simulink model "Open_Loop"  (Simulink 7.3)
settings: Solver=ode45  StartTime=0.0  StopTime=30  RelTol=1e-3
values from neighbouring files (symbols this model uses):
  d2r = pi/180    (= 0.0174532925199)    [start.m]    (also in Pl.m; run.m; pl.m)
  Ka = (1+2*zeta*lamb)*Jgi*wcmg^2    (= 292500)    [start.m]
  Kb = (2*zeta+lamb)*wcmg/Ka    (= 0.00410256410256)    [start.m]
  ki = 0.07    [start.m]
  Kii = lamb*Jgi*wcmg^3    (= 37500000)    [start.m]
  kp = 7.3    [start.m]
  r2d = 180/pi    (= 57.2957795131)    [start.m]    (also in Pl.m; run.m; pl.m)
undefined symbols (not defined in the file or in its folder): Af, Bf, Cf, Df, Lin_Steering, Tglim

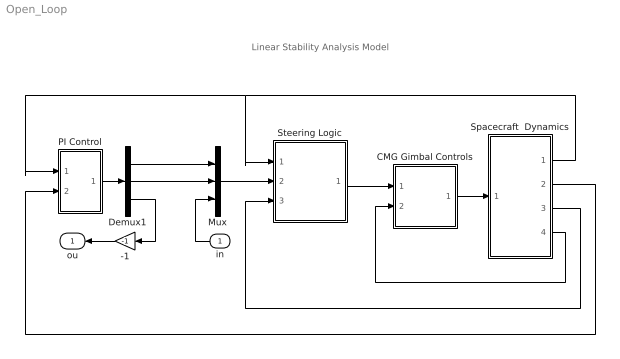
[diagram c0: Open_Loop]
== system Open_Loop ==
  note: Linear Stability Analysis Model
  in : Inport
  -1 : Gain  Gain=-1  ParameterDataType=sfix(16)  ParameterScaling=2^0  OutDataType=sfix(16)  OutScaling=2^0
  CMG Gimbal Controls : Subsystem
  Demux1 : Demux  Outputs=3
  Mux : Mux  Inputs=3
  PI Control : Subsystem
  Spacecraft  Dynamics : Subsystem
  Steering Logic : Subsystem
  ou : Outport
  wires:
  CMG Gimbal Controls/1(Tc) -> Spacecraft  Dynamics/1(Tc)
  Spacecraft  Dynamics/4(deldot) -> CMG Gimbal Controls/2(deldot)
  Steering Logic/1(deldot) -> CMG Gimbal Controls/1(deldc)
  Spacecraft  Dynamics/1(rate) -> Steering Logic/1(wb), PI Control/1(wb)
  Spacecraft  Dynamics/3(delta) -> Steering Logic/3(delta)
  Spacecraft  Dynamics/2(atti) -> PI Control/2(ater)
  Mux/1 -> Steering Logic/2(we)
  PI Control/1(wer) -> Demux1/1
  -1/1 -> ou/1
  Demux1/1 -> Mux/1
  Demux1/2 -> Mux/2
  Demux1/3 -> -1/1
  in/1 -> Mux/3

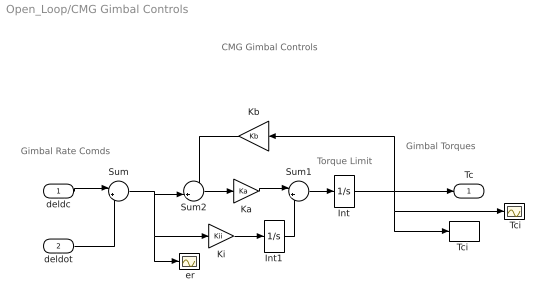
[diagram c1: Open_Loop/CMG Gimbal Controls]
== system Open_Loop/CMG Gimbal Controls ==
  note: Gimbal Rate Comds
  note: CMG Gimbal Controls
  note: Torque Limit
  note: Gimbal Torques
  deldc : Inport  PortDimensions=4  OutDataType=sfix(16)  OutScaling=2^0
  deldot : Inport  Port=2  PortDimensions=4  OutDataType=sfix(16)  OutScaling=2^0
  " Tci" : Scope
  " er" : Scope
  Int : Integrator  UpperSaturationLimit=[1 1 1 1]*Tglim  LowerSaturationLimit=-[1 1 1 1]*Tglim
  Int1 : Integrator  UpperSaturationLimit=0  LowerSaturationLimit=0
  Ka : Gain  Gain=Ka  ParameterDataType=sfix(16)  ParameterScaling=2^0  OutDataType=sfix(16)  OutScaling=2^0
  Kb : Gain  Gain=Kb  ParameterDataType=sfix(16)  ParameterScaling=2^0  OutDataType=sfix(16)  OutScaling=2^0
  Ki : Gain  Gain=Kii  ParameterDataType=sfix(16)  ParameterScaling=2^0  OutDataType=sfix(16)  OutScaling=2^0
  Sum : Sum  Inputs=|+-  OutDataType=sfix(16)  OutScaling=2^0
  Sum1 : Sum  Inputs=|++  OutDataType=sfix(16)  OutScaling=2^0
  Sum2 : Sum  Inputs=-+|  OutDataType=sfix(16)  OutScaling=2^0
  "Tci " : ToWorkspace  VariableName=Tci  SampleTime=-1  SaveFormat=Array
  Tc : Outport  OutDataType=sfix(16)  OutScaling=2^0
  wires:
  deldot/1 -> Sum/2
  deldc/1 -> Sum/1
  Sum/1 -> " er"/1, Ki/1, Sum2/2
  Kb/1 -> Sum2/1
  Int1/1 -> Sum1/2
  Ki/1 -> Int1/1
  Sum1/1 -> Int/1
  Ka/1 -> Sum1/1
  Sum2/1 -> Ka/1
  Int/1 -> Tc/1, " Tci"/1, "Tci "/1, Kb/1

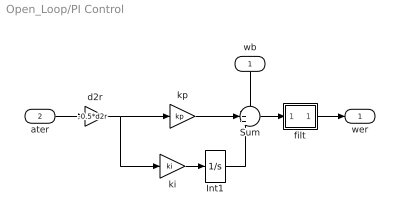
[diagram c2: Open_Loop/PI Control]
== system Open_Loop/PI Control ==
  wb : Inport
  ater : Inport  Port=2
  Int1 : Integrator  UpperSaturationLimit=0  LowerSaturationLimit=0
  Sum : Sum  Inputs=-++  OutDataType=sfix(16)  OutScaling=2^0
  d2r : Gain  Gain=-0.5*d2r  ParameterDataType=sfix(16)  ParameterScaling=2^0  OutDataType=sfix(16)  OutScaling=2^0
  filt : Subsystem
  ki : Gain  Gain=ki  ParameterDataType=sfix(16)  ParameterScaling=2^0  OutDataType=sfix(16)  OutScaling=2^0
  kp : Gain  Gain=kp  ParameterDataType=sfix(16)  ParameterScaling=2^0  OutDataType=sfix(16)  OutScaling=2^0
  wer : Outport
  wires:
  ater/1 -> d2r/1
  kp/1 -> Sum/2
  ki/1 -> Int1/1
  Int1/1 -> Sum/3
  wb/1 -> Sum/1
  Sum/1 -> filt/1(in)
  d2r/1 -> ki/1, kp/1
  filt/1(ou) -> wer/1

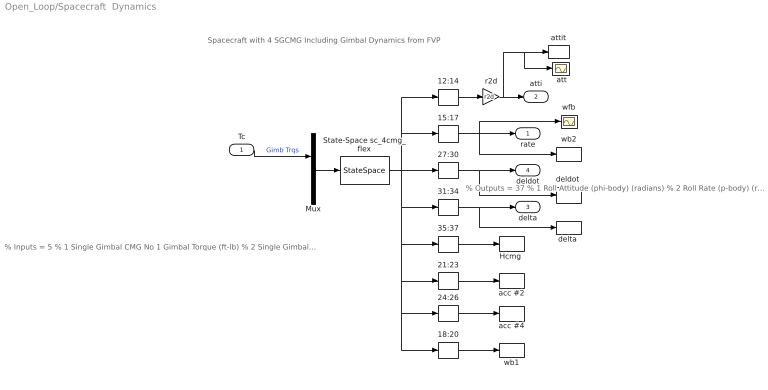
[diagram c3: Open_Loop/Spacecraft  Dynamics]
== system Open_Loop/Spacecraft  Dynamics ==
  note: % Outputs = 37 % 1 Roll Attitude (phi-body) (radians) % 2 Roll Rate (p-body) (rad/sec) % 3 Pitch Attitude (thet-bdy) (radians) % 4 Pitch Rate (q-body) (rad/sec) % 5 Yaw Attitude (psi-body) (radians) % 6 Yaw Rate (r-body) (rad/sec) % 7 Angle of attack, alfa, (radians) % 8 Angle of sideslip, beta, (radian) % 9 Change in Altitude, delta-h, (feet) % 10 Forward Acceleration (V-dot) (ft/sec) % 11 Cross Range Velocity (Vcr) (ft/sec) % 12 Gyro # 1, Roll Attitude (Body) (radians) % 13 Gyro # 2, Pitch Attitude (Body) (radians) % 14 Gyro # 3, Yaw Attitude (Body) (radians) % 15 Rate-Gyro # 4, Roll Rate (Body) (rad/sec) % 16 Rate-Gyro # 5, Pitch Rate (Body) (rad/sec) % 17 Rate-Gyro # 6, Yaw Rate (Body) (rad/sec) % 18 Rate-Gyro # 7, Roll Rate (Body) (rad/sec) % 19 Rate-Gyro # 8, Pitch Rate (Body) (rad/sec) % 20 Rate-Gyro # 9, Yaw Rate (Body) (rad/sec) % 21 Accelerom # 1, (along X), (ft/sec^2) Translat. Acceler % 22 Accelerom # 2, (along Y), (ft/sec^2) Translat. Acceler % 23 Accelerom # 3, (along Z), (ft/sec^2) Translat. Acceler % 24 Accelerom # 4, (along X), (ft/sec^2) Translat. Acceler % 25 Accelerom # 5, (along Y), (ft/sec^2) Translat. Acceler % 26 Accelerom # 6, (along Z), (ft/sec^2) Translat. Acceler % 27 SGCMG # 1 Gimbal Rate (rad/sec) % 28 SGCMG # 2 Gimbal Rate (rad/sec) % 29 SGCMG # 3 Gimbal Rate (rad/sec) % 30 SGCMG # 4 Gimbal Rate (rad/sec) % 31 SGCMG # 1 Gimbal Angle (radian) % 32 SGCMG # 2 Gimbal Angle (radian) % 33 SGCMG # 3 Gimbal Angle (radian) % 34 SGCMG # 4 Gimbal Angle (radian) % 35 SGCMG Array Momentum in X-axis (ft-lb-sec) % 36 SGCMG Array Momentum in Y-axis (ft-lb-sec) % 37 SGCMG Array Momentum in Z-axis (ft-lb-sec)
  note: % Inputs = 5 % 1 Single Gimbal CMG No 1 Gimbal Torque (ft-lb) % 2 Single Gimbal CMG No 2 Gimbal Torque (ft-lb) % 3 Single Gimbal CMG No 3 Gimbal Torque (ft-lb) % 4 Single Gimbal CMG No 4 Gimbal Torque (ft-lb) % 5 Ext Force Direct. = (1.0000 0.0000 0.0000)
  note: Spacecraft with 4 SGCMG Including Gimbal Dynamics from FVP
  Tc : Inport  PortDimensions=4  OutDataType=sfix(16)  OutScaling=2^0
  " att" : Scope
  " wfb " : Scope
  12:14 : Selector  InputPortWidth=37  IndexOptions=Index vector (dialog)  Indices=[12:14]  OutputSizes=1
  15:17 : Selector  InputPortWidth=37  IndexOptions=Index vector (dialog)  Indices=[15:17]  OutputSizes=1
  18:20 : Selector  InputPortWidth=37  IndexOptions=Index vector (dialog)  Indices=[18:20]  OutputSizes=1
  21:23 : Selector  InputPortWidth=37  IndexOptions=Index vector (dialog)  Indices=[21:23]  OutputSizes=1
  24:26 : Selector  InputPortWidth=37  IndexOptions=Index vector (dialog)  Indices=[24:26]  OutputSizes=1
  27:30 : Selector  InputPortWidth=37  IndexOptions=Index vector (dialog)  Indices=[27:30]  OutputSizes=1
  31:34 : Selector  InputPortWidth=37  IndexOptions=Index vector (dialog)  Indices=[31:34]  OutputSizes=1
  35:37 : Selector  InputPortWidth=37  IndexOptions=Index vector (dialog)  Indices=[35:37]  OutputSizes=1
  "Hcmg " : ToWorkspace  VariableName=Hcmg  SampleTime=-1  SaveFormat=Array
  Mux : Mux  Inputs="[4,  1]"
  State-Space sc_4cmg_flex : StateSpace  A=Af  B=Bf  C=Cf  D=Df
  acc #2 : ToWorkspace  VariableName=acc_2  SampleTime=-1  SaveFormat=Array
  acc #4 : ToWorkspace  VariableName=acc_4  SampleTime=-1  SaveFormat=Array
  attit : ToWorkspace  VariableName=atti  SampleTime=-1  SaveFormat=Array
  "deldot " : ToWorkspace  VariableName=deld  SampleTime=-1  SaveFormat=Array
  "delta " : ToWorkspace  VariableName=delta  SampleTime=-1  SaveFormat=Array
  r2d : Gain  Gain=r2d  ParameterDataType=sfix(16)  ParameterScaling=2^0  OutDataType=sfix(16)  OutScaling=2^0
  wb1 : ToWorkspace  VariableName=wb_1  SampleTime=-1  SaveFormat=Array
  wb2 : ToWorkspace  VariableName=wb_2  SampleTime=-1  SaveFormat=Array
  rate : Outport  OutDataType=sfix(16)  OutScaling=2^0
  atti : Outport  Port=2  OutDataType=sfix(16)  OutScaling=2^0
  delta : Outport  Port=3  OutDataType=sfix(16)  OutScaling=2^0
  deldot : Outport  Port=4  OutDataType=sfix(16)  OutScaling=2^0
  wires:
  24:26/1 -> acc #4/1
  21:23/1 -> acc #2/1
  18:20/1 -> wb1/1
  r2d/1 -> " att"/1, attit/1, atti/1
  35:37/1 -> "Hcmg "/1
  31:34/1 -> "delta "/1, delta/1
  27:30/1 -> "deldot "/1, deldot/1
  15:17/1 -> " wfb "/1, wb2/1, rate/1
  12:14/1 -> r2d/1
  State-Space sc_4cmg_flex/1 -> 24:26/1, 18:20/1, 21:23/1, 35:37/1, 31:34/1, 27:30/1, 15:17/1, 12:14/1
  Tc/1 -> Mux/1  "Gimb Trqs"
  Mux/1 -> State-Space sc_4cmg_flex/1

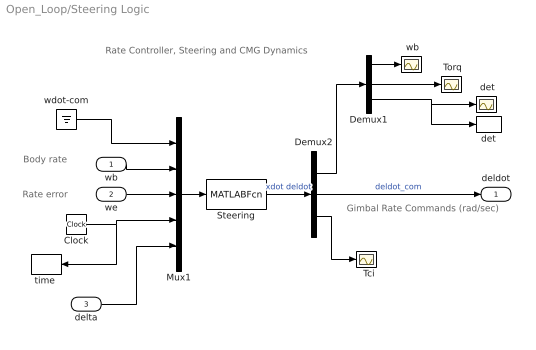
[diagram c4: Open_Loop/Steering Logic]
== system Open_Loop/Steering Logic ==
  note: Body rate
  note: Rate error
  note: Gimbal Rate Commands (rad/sec)
  note: Rate Controller, Steering and CMG Dynamics
  wb : Inport  PortDimensions=3  OutDataType=sfix(16)  OutScaling=2^0
  we : Inport  Port=2  PortDimensions=3  OutDataType=sfix(16)  OutScaling=2^0
  delta : Inport  Port=3  OutDataType=sfix(16)  OutScaling=2^0
  "  Tci" : Scope
  " Torq" : Scope
  " det" : Scope
  " wb" : Scope
  Clock : Clock
  Demux1 : Demux  Outputs=3
  Demux2 : Demux  Outputs=[3,4,4]
  Mux1 : Mux  Inputs=[3,3,3, 1,4]
  Steering : MATLABFcn  MATLABFcn=Lin_Steering( u(1:3), u(4:6), u(7:9), u(10), u(11:14) )  OutputDimensions=11
  det : ToWorkspace  VariableName=det  SampleTime=-1  SaveFormat=Array
  "time " : ToWorkspace  VariableName=time  SampleTime=-1  SaveFormat=Array
  wdot-com : Ground
  deldot : Outport  OutDataType=sfix(16)  OutScaling=2^0
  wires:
  Demux2/3 -> "  Tci"/1
  delta/1 -> Mux1/5
  Mux1/1 -> Steering/1
  we/1 -> Mux1/3
  Demux1/2 -> " Torq"/1
  Demux1/3 -> det/1, " det"/1
  Demux1/1 -> " wb"/1
  Clock/1 -> "time "/1, Mux1/4
  wb/1 -> Mux1/2
  Demux2/1 -> Demux1/1
  Demux2/2 -> deldot/1  "deldot_com"
  Steering/1 -> Demux2/1  "xdot deldot"
  wdot-com/1 -> Mux1/1

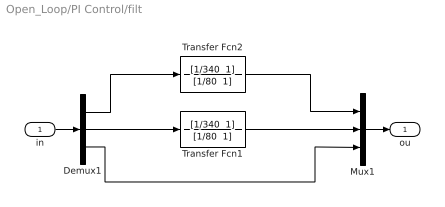
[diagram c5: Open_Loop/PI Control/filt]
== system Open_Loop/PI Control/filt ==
  in : Inport  OutDataType=sfix(16)  OutScaling=2^0
  Demux1 : Demux  Outputs=3
  Mux1 : Mux  Inputs=3
  Transfer Fcn1 : TransferFcn  Numerator="[1/340  1]"  Denominator="[1/80  1]"
  Transfer Fcn2 : TransferFcn  Numerator="[1/340  1]"  Denominator="[1/80  1]"
  ou : Outport  OutDataType=sfix(16)  OutScaling=2^0
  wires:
  Demux1/1 -> Transfer Fcn2/1
  Demux1/2 -> Transfer Fcn1/1
  Demux1/3 -> Mux1/3
  in/1 -> Demux1/1
  Mux1/1 -> ou/1
  Transfer Fcn2/1 -> Mux1/1
  Transfer Fcn1/1 -> Mux1/2
